(* Logix 5000 AddOnInstructionDefinition export OPCE1WIE_ACDC_Drive_Profile; software revision 19.01 *)

ADD_ON_INSTRUCTION OPCE1WIE_ACDC_Drive_Profile   (* revision 1.0 *)
// Interface for AC/DC Drive Profile that uses Input Assembly Instance 71 and Output Assembly Instance 21.
VAR_IN_OUT
   I_Data : INT[2]; {required}   // Input data
   O_Data : INT[2]; {required}   // Output data
END_VAR
VAR_INPUT
   RunForward : BOOL; {required}   // Run forward
   RunReverse : BOOL; {required}   // Run reverse
   ResetFault : BOOL; {required}   // Reset fault
   SpeedReference : INT; {access Read Only, required}   // Speed reference (RPM)
END_VAR
VAR_OUTPUT
   Faulted : BOOL; {access Read Only, visible}   // Faulted
   RunningForward : BOOL; {access Read Only, visible}   // Running forward
   RunningReverse : BOOL; {access Read Only, visible}   // Running reverse
   Ready : BOOL; {access Read Only, visible}   // Ready
   AtReference : BOOL; {access Read Only, visible}   // Up-to-speed
   DriveState : SINT; {access Read Only, visible}   // Drive state (0 = vendor specific, 1 = startup, 2 = not ready, 3 = ready, 4 = enabled, 5 = stopping, 6 = fault stop, 7 = faulted)
   SpeedActual : INT; {access Read Only, visible}   // Actual speed (RPM)
END_VAR
VAR
   temp : INT; {access None}
END_VAR

ROUTINE Logic   (* ladder *)
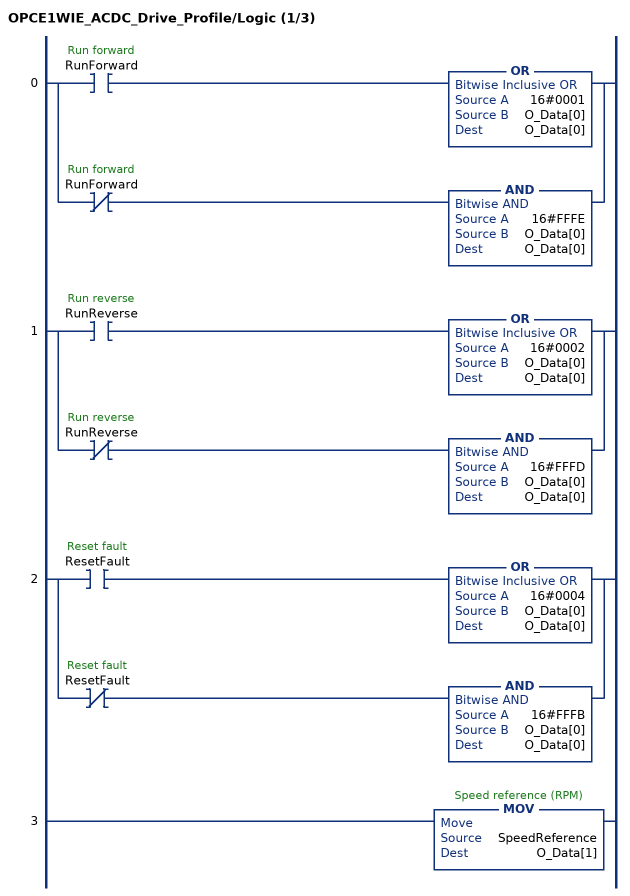
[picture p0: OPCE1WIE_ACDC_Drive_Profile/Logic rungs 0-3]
   0: [XIC(RunForward) OR(16#0001,O_Data[0],O_Data[0]) ,XIO(RunForward) AND(16#FFFE,O_Data[0],O_Data[0]) ];
   1: [XIC(RunReverse) OR(16#0002,O_Data[0],O_Data[0]) ,XIO(RunReverse) AND(16#FFFD,O_Data[0],O_Data[0]) ];
   2: [XIC(ResetFault) OR(16#0004,O_Data[0],O_Data[0]) ,XIO(ResetFault) AND(16#FFFB,O_Data[0],O_Data[0]) ];
   3: MOV(SpeedReference,O_Data[1]);
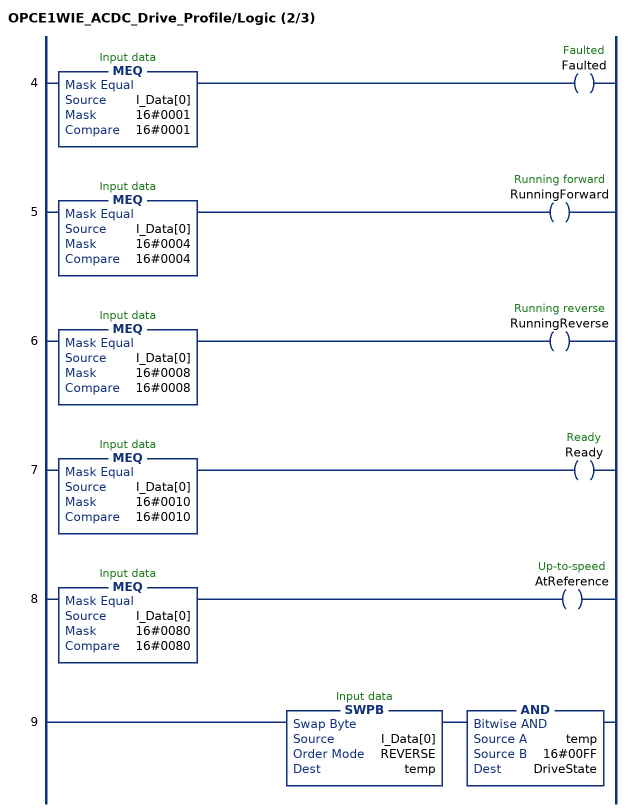
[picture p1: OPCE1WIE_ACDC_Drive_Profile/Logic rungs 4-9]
   4: MEQ(I_Data[0],16#0001,16#0001)OTE(Faulted);
   5: MEQ(I_Data[0],16#0004,16#0004)OTE(RunningForward);
   6: MEQ(I_Data[0],16#0008,16#0008)OTE(RunningReverse);
   7: MEQ(I_Data[0],16#0010,16#0010)OTE(Ready);
   8: MEQ(I_Data[0],16#0080,16#0080)OTE(AtReference);
   9: SWPB(I_Data[0],REVERSE,temp)AND(temp,16#00FF,DriveState);
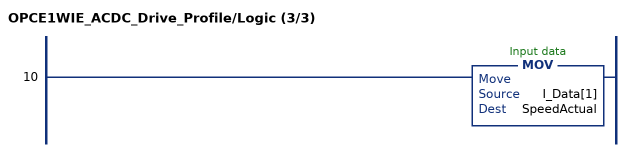
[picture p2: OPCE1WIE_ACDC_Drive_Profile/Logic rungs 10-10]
   10: MOV(I_Data[1],SpeedActual);
END_ROUTINE
END_ADD_ON_INSTRUCTION
